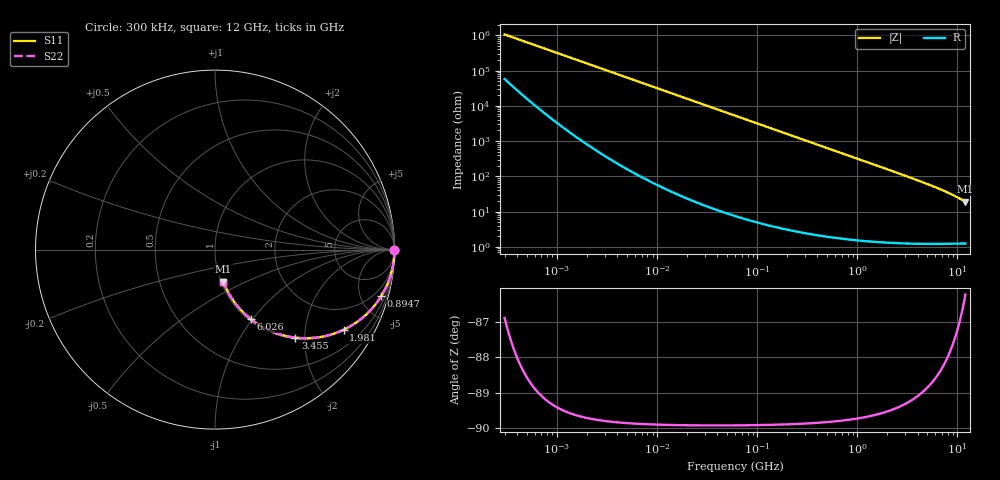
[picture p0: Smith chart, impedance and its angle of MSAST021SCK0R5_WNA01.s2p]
! MSAST021SCK0R5_WNA01  S-PARAMETER MODEL  ( General Type )
! Model Generated by TAIYO YUDEN Corporation (http://www.ty-top.com)
! Version 2.0
! TAIYO YUDEN Control No. 181101
! Copyright(c) 2015 TAIYO YUDEN CO.,LTD. All Rights Reserved.
! Product Description (link to TY-COMPAS)
! https://ds.yuden.co.jp/TYCOMPAS/or/detail?pn=MSAST021SCK0R5BWNA01&u=M
! Products Name : Multilayer Ceramic Capacitors
! Characteristics :
!  Capacitance : 0.5 pF , Rated Voltage : 25V , TCC : CK / C0K
!  Case Size : 0.25 x 0.125 / 0.0098 x 0.0049 [mm/inch] , Thickness : 0.125 / 0.0049 [mm/inch]
!  (Conditions: Temperature = 25 degC , DC Bias Current/Voltage = 0A / 0V)
! External Node Assignments :
!  1  o---| |---o  2
! GND o---------o GND
! Frequency Range : 0.3MHz  -  12000MHz  [ 401 STEP ]
# MHz S RI R 50
! Freq[MHz].  S11 Real  S11 Imag  S21 Real  S21 Imag  S12 Real  S12 Imag  S22 Real  S22 Imag
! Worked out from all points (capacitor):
!   401 points, 300 kHz to 12 GHz, reference 50 ohm
!   read as one part in series: C = 500 fF near 316.3 kHz
!   lowest |Z| = 18.9 ohm at 12 GHz (marker M1)
!   S11 on the Smith chart (normalised r, x): 300 kHz: open; 894.7 MHz: 1.03, -7.10; 1.981 GHz: 1.03, -3.19; 3.455 GHz: 1.02, -1.80; 6.026 GHz: 1.02, -0.98; 12 GHz: 1.02, -0.38
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0.3  1 -9.4e-05  5.11e-06 9.4e-05  5.11e-06 9.4e-05  1 -9.4e-05
0.316324  1 -9.91e-05  4.95e-06 9.91e-05  4.95e-06 9.91e-05  1 -9.91e-05
0.342489  1 -0.000107  4.73e-06 0.000107  4.73e-06 0.000107  1 -0.000107
1.769972  1 -0.000556  3.44e-06 0.000556  3.44e-06 0.000556  1 -0.000556
10.44266  1 -0.00328  1.65e-05 0.00328  1.65e-05 0.00328  1 -0.00328
60  0.9996 -0.0188  0.000382 0.0188  0.000382 0.0188  0.9996 -0.0188
164.1901  0.9973 -0.0514  0.00275 0.0514  0.00275 0.0514  0.9973 -0.0514
353.9943  0.9875 -0.1098  0.0125 0.1098  0.0125 0.1098  0.9875 -0.1098
570.2811  0.9683 -0.1735  0.0317 0.1735  0.0317 0.1735  0.9683 -0.1735
894.6982  0.9256 -0.2603  0.0744 0.2603  0.0744 0.2603  0.9256 -0.2603
1105.905  0.8906 -0.3096  0.1094 0.3096  0.1094 0.3096  0.8906 -0.3096
1366.97  0.8418 -0.3619  0.1582 0.3619  0.1582 0.3619  0.8418 -0.3619
1645.489  0.7857 -0.4069  0.2143 0.4069  0.2143 0.4069  0.7857 -0.4069
1980.756  0.7161 -0.4468  0.2839 0.4468  0.2839 0.4468  0.7161 -0.4468
2088.533  0.6938 -0.4566  0.3062 0.4566  0.3062 0.4566  0.6938 -0.4566
2722.03  0.5695 -0.4897  0.4305 0.4897  0.4305 0.4897  0.5695 -0.4897
3454.93  0.4479 -0.4905  0.5521 0.4905  0.5521 0.4905  0.4479 -0.4905
4502.883  0.3181 -0.4569  0.6819 0.4569  0.6819 0.4569  0.3181 -0.4569
6026.253  0.1994 -0.3874  0.8006 0.3874  0.8006 0.3874  0.1994 -0.3874
7064.448  0.1486 -0.3411  0.8514 0.3411  0.8514 0.3411  0.1486 -0.3411
8503.825  0.1019 -0.284  0.8981 0.284  0.8981 0.284  0.1019 -0.284
12000  0.0454 -0.1779  0.9546 0.1779  0.9546 0.1779  0.0454 -0.1779
